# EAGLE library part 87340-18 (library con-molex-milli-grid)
RECEPTACAL
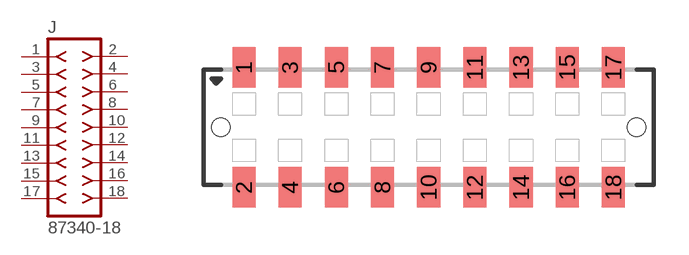
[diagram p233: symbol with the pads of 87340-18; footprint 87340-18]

Designator prefix J

## 87340-18  [87340-18]
1  1  pas
2  2  pas
3  3  pas
4  4  pas
5  5  pas
6  6  pas
7  7  pas
8  8  pas
9  9  pas
10  10  pas
11  11  pas
12  12  pas
13  13  pas
14  14  pas
15  15  pas
16  16  pas
17  17  pas
18  18  pas

## Footprint 87340-18 (pad centres in mm)
RECEPTACAL SMD Dual Row, Vertical, Low Profile
smd 1 x 1.75: 1 -8,2.6; 2 -8,-2.6; 3 -6,2.6; 4 -6,-2.6; 5 -4,2.6; 6 -4,-2.6; 7 -2,2.6; 8 -2,-2.6; 9 0,2.6; 10 0,-2.6; 11 2,2.6; 12 2,-2.6; 13 4,2.6; 14 4,-2.6; 15 6,2.6; 16 6,-2.6; 17 8,2.6; 18 8,-2.6
hole 0.8 at -9,0
hole 0.8 at 9,0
